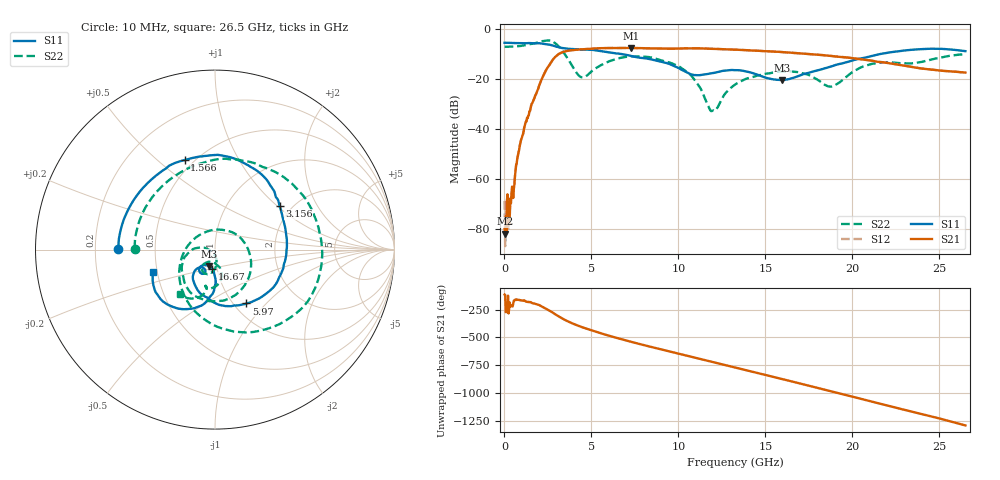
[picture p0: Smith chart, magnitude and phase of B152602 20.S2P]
!  2-Port S-parameters saved by WinCal
! VAR MeasName=S-Parameters (CALIBRATED_DATA) read from VNA (N5242A)
! VAR MeasDate=2016-1-5 16:28:13
! VAR NAME=B152602 20
! VAR FILENAME=B152602 20.S2P
! VAR DATE=2016-1-5 16:28:13
! VAR PHYS_PORTS=1,2
# Hz S DB R 50
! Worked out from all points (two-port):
!   801 points, 10 MHz to 26.5 GHz, reference 50 ohm
!   highest |S21| = -7.43 dB at 7.262 GHz (marker M1); lowest = -81.7 dB at 43.11 MHz (marker M2)
!   |S21| within 3 dB of the highest: 3.027 GHz to 18.46 GHz (15.43 GHz wide, 144 % of centre)
!   lowest |S11| = -20.3 dB at 15.97 GHz (marker M3), VSWR 1.21, Z = 46 - j8.42 ohm
!   |S11| at or under -10 dB: 6.83 GHz to 21.51 GHz (14.68 GHz wide, 104 % of centre)
!   |S22| runs from -32.7 to -4.4 dB; largest |S21 - S12| = 0.003
!   S11 on the Smith chart (normalised r, x): 10 MHz: 0.30, +0.00; 1.566 GHz: 0.45, +0.62; 3.156 GHz: 1.73, +1.04; 5.97 GHz: 1.14, -0.78; 16.67 GHz: 0.95, -0.21; 26.5 GHz: 0.48, -0.14
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1e7  -5.38 179.5  -79.73 -114.3  -68.62 -117.0  -6.97 179.3
4.31125e7  -5.37 178.0  -81.71 -117.6  -86.70 103.0  -6.97 177.4
1.755625e8  -5.38 171.8  -65.97 84.4  -66.08 81.5  -6.95 169.2
3.41125e8  -5.42 164.3  -67.59 134.8  -69.69 130.5  -6.93 159.0
8.70925e8  -5.54 140.6  -46.94 -162.5  -46.88 -162.3  -6.70 126.0
1.566288e9  -5.56 108.7  -29.83 171.2  -29.84 171.3  -5.80 78.2
2.460325e9  -6.01 65.1  -15.49 110.9  -15.49 110.9  -4.47 -1.8
3.155688e9  -7.23 34.2  -9.74 45.0  -9.75 45.0  -7.09 -84.7
3.652375e9  -7.76 17.1  -8.57 3.5  -8.58 3.5  -11.85 -140.6
4.447075e9  -8.10 -10.6  -8.02 -47.5  -8.01 -47.4  -19.20 110.5
5.97025e9  -9.18 -59.7  -7.48 -123.6  -7.46 -123.7  -12.93 -27.5
7.261638e9  -10.60 -91.1  -7.43 -179.5  -7.42 -179.5  -10.81 -81.2
8.851038e9  -12.72 -117.9  -7.66 117.3  -7.63 117.2  -12.05 -132.8
1.067222e10  -17.87 -130.0  -7.60 48.6  -7.57 48.6  -18.02 179.8
1.19305e10  -17.52 -114.0  -7.81 -0.9  -7.79 -1.1  -32.66 -141.7
1.3255e10  -16.32 -121.4  -8.14 -51.6  -8.12 -51.8  -22.10 -83.7
1.597022e10  -20.28 -110.5  -9.12 -156.4  -9.09 -156.3  -16.88 -109.0
1.666559e10  -19.26 -97.4  -9.47 177.0  -9.42 176.9  -16.93 -117.6
1.769208e10  -16.97 -91.0  -9.96 136.9  -9.93 137.0  -18.94 -127.3
1.88179e10  -14.78 -88.9  -10.67 92.5  -10.68 92.5  -22.86 -99.2
2.209604e10  -9.29 -108.7  -13.55 -37.9  -13.47 -38.1  -13.18 -100.9
2.65e10  -8.72 -159.9  -17.30 145.7  -17.30 145.4  -9.99 -128.0
